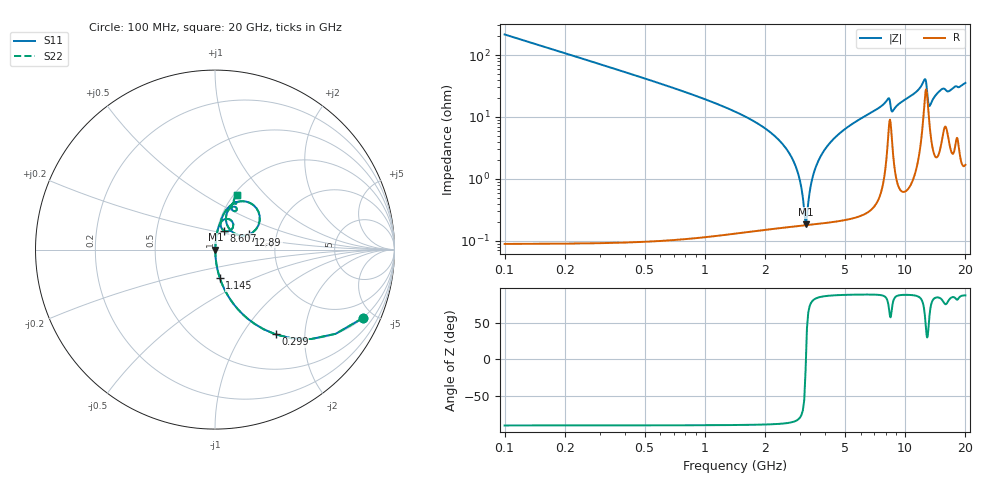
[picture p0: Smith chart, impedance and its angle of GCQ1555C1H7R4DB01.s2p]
!Murata Part Number: GCQ1555C1H7R4DB01
!These Parameters are Measured in Series Mode Connection
!Data Generated on Mar 13, 2026
!  o--ll--o
!Port1  Port2
!  o------o
!Operation Temp=25[degC], DC Bias Voltage=0[V]
!Freq. Start=100[MHz] Stop=20[GHz] 401[Steps]
# Hz S RI R 50
!Freq.(Hz) S11(Real) S11(Imag) S21(Real) S21(Imag) S12(Real) S12(Imag) S22(Real) S22(Imag)
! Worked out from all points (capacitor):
!   401 points, 100 MHz to 20 GHz, reference 50 ohm
!   read as one part in series: C = 7.4 pF near 199.5 MHz
!   lowest |Z| = 184 mohm at 3.184 GHz (marker M1)
!   series resonance near 3.195 GHz, so ESL is about 340 pH
!   S11 on the Smith chart (normalised r, x): 100 MHz: 1.00, -4.30; 299 MHz: 1.00, -1.43; 1.145 GHz: 1.00, -0.33; 8.607 GHz: 1.08, +0.23; 12.89 GHz: 1.44, +0.25; 20 GHz: 1.03, +0.71
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1e8  0.8219 -0.3824  0.1781 0.3824  0.1781 0.3824  0.8219 -0.3824
2.99e8  0.3372 -0.4721  0.6628 0.4721  0.6628 0.4721  0.3372 -0.4721
5.975e8  0.1083 -0.3093  0.8917 0.3093  0.8917 0.3093  0.1083 -0.3093
1.14475e9  0.0272 -0.159  0.9728 0.159  0.9728 0.159  0.0272 -0.159
2.5875e9  0.00247 -0.0285  0.9975 0.0285  0.9975 0.0285  0.00247 -0.0285
2.886e9  0.00191 -0.0137  0.9981 0.0137  0.9981 0.0137  0.00191 -0.0137
3.1845e9  0.00178 -0.000453  0.9982 0.000453  0.9982 0.000453  0.00178 -0.000453
3.284e9  0.00182 0.00369  0.9982 -0.00369  0.9982 -0.00369  0.00182 0.00369
3.43325e9  0.00193 0.00969  0.9981 -0.00969  0.9981 -0.00969  0.00193 0.00969
3.7815e9  0.00242 0.0229  0.9976 -0.0229  0.9976 -0.0229  0.00242 0.0229
4.3785e9  0.0039 0.0434  0.9961 -0.0434  0.9961 -0.0434  0.0039 0.0434
6.7665e9  0.0167 0.1154  0.9833 -0.1154  0.9833 -0.1154  0.0167 0.1154
8.20925e9  0.0722 0.1709  0.9278 -0.1709  0.9278 -0.1709  0.0722 0.1709
8.60725e9  0.0501 0.1059  0.9499 -0.1059  0.9499 -0.1059  0.0501 0.1059
1.005e10  0.0415 0.1837  0.9585 -0.1837  0.9585 -0.1837  0.0415 0.1837
1.2438e10  0.2044 0.2548  0.7956 -0.2548  0.7956 -0.2548  0.2044 0.2548
1.288575e10  0.1884 0.0842  0.8116 -0.0842  0.8116 -0.0842  0.1884 0.0842
1.31345e10  0.1021 0.0945  0.8979 -0.0945  0.8979 -0.0945  0.1021 0.0945
1.338325e10  0.07 0.132  0.93 -0.132  0.93 -0.132  0.07 0.132
1.497525e10  0.0904 0.2352  0.9096 -0.2352  0.9096 -0.2352  0.0904 0.2352
1.67165e10  0.0921 0.2316  0.9079 -0.2316  0.9079 -0.2316  0.0921 0.2316
2e10  0.1233 0.3059  0.8767 -0.3059  0.8767 -0.3059  0.1233 0.3059
